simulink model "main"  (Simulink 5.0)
settings: Solver=FixedStepDiscrete  StartTime=0.0  StopTime=10.0  FixedStep=Ts  RelTol=1e-3

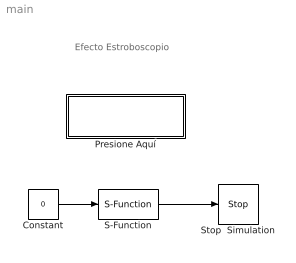
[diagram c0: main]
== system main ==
  note: Efecto Estroboscopio
  Constant : Constant  Value=0
  Presione Aquí : Subsystem
  S-Function : S-Function  FunctionName=circulo  Parameters=Ts
  Stop  Simulation : Stop
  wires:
  Constant/1 -> S-Function/1
  S-Function/1 -> Stop  Simulation/1

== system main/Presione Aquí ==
